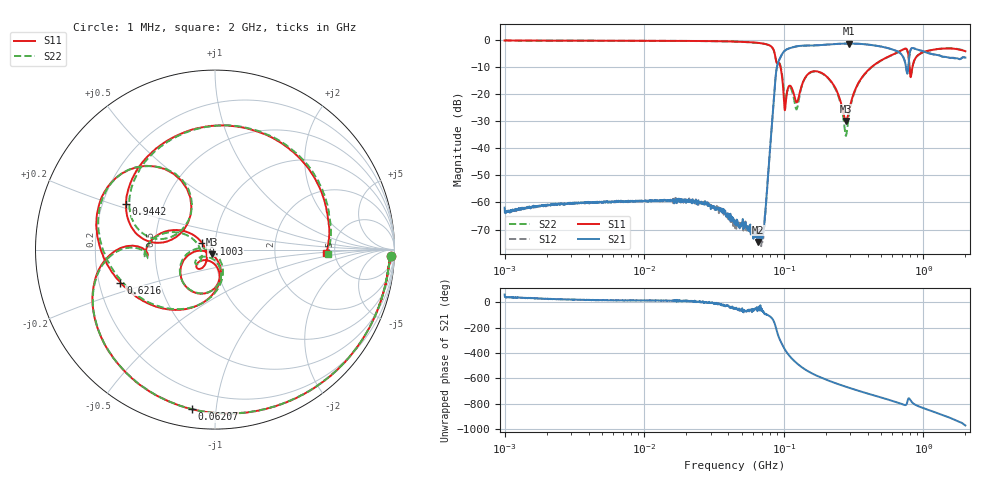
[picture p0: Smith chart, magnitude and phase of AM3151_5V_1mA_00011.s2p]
! Date/Time: Fri Jun 26 10:26:44 2020
! Network Analyzer:  Rev:
! Sweep from 1000000.0 to 2000000000.0, 1601 Points ! Power Supply: 0 V, 0 A
# HZ S DB R 50
!freq MagS11 AngS11 MagS21 AngS21 MagS12 AngS12 MagS22 AngS22
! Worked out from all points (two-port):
!   1601 points, 1 MHz to 2 GHz, reference 50 ohm
!   highest |S21| = -1.29 dB at 294.8 MHz (marker M1); lowest = -74.6 dB at 65.71 MHz (marker M2)
!   |S21| within 3 dB of the highest: 99.97 MHz to 657.4 MHz (557.4 MHz wide, 147 % of centre); 803 MHz to 1.012 GHz (208.6 MHz wide, 23 % of centre)
!   lowest |S11| = -29.9 dB at 279.8 MHz (marker M3), VSWR 1.07, Z = 48.3 - j2.64 ohm
!   |S11| at or under -10 dB: 94.74 MHz to 425.1 MHz (330.4 MHz wide, 127 % of centre); 796 MHz to 835 MHz (39.01 MHz wide, 4.78 % of centre)
!   |S22| runs from -35.4 to -0.2 dB; largest |S21 - S12| = 0.01
!   S11 on the Smith chart (normalised r, x): 1 MHz: 24, -45; 62.07 MHz: 0.09, -0.86; 100.3 MHz: 0.87, +0.06; 621.6 MHz: 0.29, -0.16; 944.2 MHz: 0.30, +0.22; 2 GHz: 4.26, -0.27
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1000000  -0.16 -2.0  -61.93 60.0  -63.38 41.0  -0.17 -2.0
3555161  -0.24 -5.5  -60.31 18.3  -60.10 18.3  -0.24 -5.5
1.263916e7  -0.29 -18.4  -59.48 11.6  -59.29 13.0  -0.29 -18.4
4.493426e7  -0.57 -67.4  -67.24 -45.5  -69.53 -48.5  -0.58 -67.4
6.206852e7  -0.93 -98.3  -71.33 -52.8  -71.77 -48.8  -0.93 -98.3
6.570964e7  -1.06 -106.0  -74.65 -61.1  -71.55 -64.4  -1.06 -106.1
7.225896e7  -1.36 -121.9  -69.16 -85.7  -69.05 -87.1  -1.37 -121.9
8.863535e7  -8.22 -179.4  -10.96 142.7  -10.96 142.8  -8.21 -177.6
1.002879e8  -22.11 153.9  -4.21 -0.3  -4.22 -0.2  -19.21 159.4
1.184292e8  -20.23 -140.8  -2.54 -101.9  -2.53 -101.9  -21.86 -150.7
1.589914e8  -11.70 -109.4  -2.01 158.7  -2.00 158.6  -11.75 -109.7
2.259679e8  -16.41 -168.0  -1.53 87.9  -1.53 87.8  -16.63 -173.4
2.798254e8  -29.95 -121.1  -1.31 52.5  -1.31 52.5  -35.21 -116.5
2.948368e8  -25.49 -80.6  -1.29 44.4  -1.29 44.3  -26.80 -66.5
3.616573e8  -13.94 -84.7  -1.46 13.5  -1.48 13.6  -14.06 -82.1
5.652395e8  -6.06 -146.0  -3.09 -49.6  -3.07 -49.7  -6.12 -147.4
6.215777e8  -5.06 -160.8  -3.75 -63.1  -3.74 -63.1  -5.14 -162.4
7.624488e8  -3.48 140.7  -12.06 -77.3  -12.06 -77.0  -3.65 137.5
8.226611e8  -12.10 167.1  -3.07 -65.3  -3.06 -65.2  -12.05 163.1
9.441749e8  -5.08 153.0  -3.77 -105.3  -3.78 -105.2  -5.14 149.5
1.400532e9  -3.14 80.2  -6.21 -172.8  -6.20 -173.0  -3.10 76.9
2e9  -4.14 -1.8  -6.50 107.9  -6.62 107.6  -4.01 -2.0
